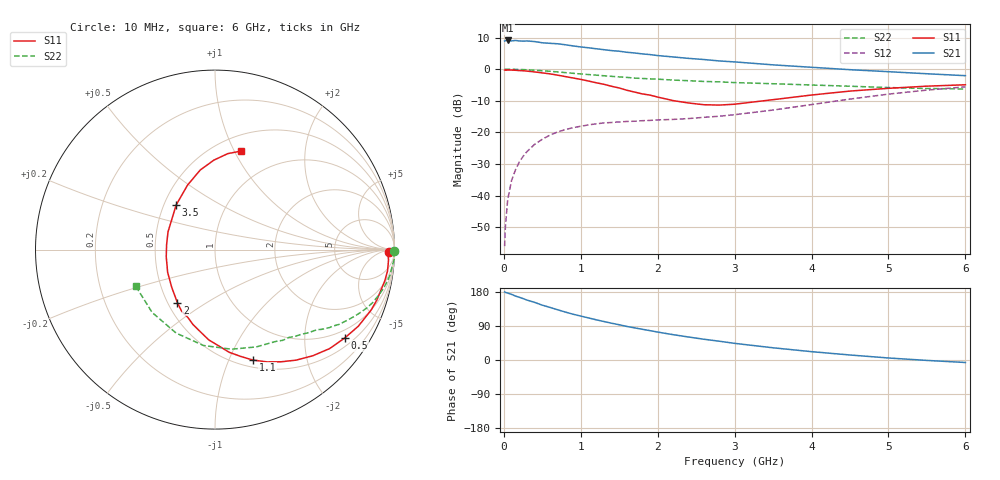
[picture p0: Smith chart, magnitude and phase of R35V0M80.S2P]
! SIEMENS Small Signal Semiconductors
! BFR181
! Si NPN RF Bipolar Junction Transistor in SOT23
! VCE = 5 V  IC = 0.8 mA
! Common Emitter S-Parameters:  May  1996
# GHz  S  MA  R  50
!  f  S11  S21  S12  S22
! GHz  MAG  ANG  MAG  ANG  MAG  ANG  MAG  ANG
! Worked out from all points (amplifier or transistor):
!   36 points, 10 MHz to 6 GHz, reference 50 ohm
!   highest |S21| = 9.1 dB at 50 MHz (marker M1)
!   |S21| within 3 dB of that: start of sweep to 1.329 GHz
!   unconditionally stable (mu >= 1): 2.149 GHz to 3.752 GHz
!   at 250 MHz: K = 0.15, MSG = 18.2 dB, |S12| = -27.6 dB
!   at 1.4 GHz: K = 0.70, MSG = 11.4 dB, |S12| = -16.8 dB
!   at 6 GHz: K = 0.89, MSG = 1.8 dB, |S12| = -5.6 dB
!   S11 on the Smith chart (normalised r, x): 10 MHz: 54, -24; 500 MHz: 0.74, -3.08; 1.1 GHz: 0.58, -1.23; 2 GHz: 0.56, -0.38; 3.5 GHz: 0.58, +0.32; 6 GHz: 0.66, +1.06
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0.01  0.9694 -0.8  2.783 179.6  0.0016 91.0  0.9982 -0.4
0.02  0.9635 -1.3  2.812 178.4  0.0032 85.2  0.9996 -0.8
0.05  0.9686 -3.4  2.844 176.6  0.0087 89.2  0.9981 -1.7
0.1  0.9685 -7.1  2.799 173.3  0.0174 85.6  0.999 -3.3
0.15  0.9619 -10.5  2.844 168.8  0.0255 82.4  0.9924 -5.1
0.2  0.9515 -13.8  2.795 165.6  0.034 80.7  0.9886 -6.7
0.3  0.9327 -21.2  2.793 158.2  0.0498 76.0  0.9782 -9.9
0.4  0.9056 -28.1  2.733 152.1  0.0649 71.7  0.9633 -13.0
0.5  0.8745 -34.3  2.613 144.7  0.0782 67.6  0.9445 -15.9
0.7  0.8045 -47.3  2.521 132.5  0.102 60.0  0.9054 -21.1
0.8  0.7641 -53.7  2.431 126.5  0.1111 56.5  0.8828 -23.4
1.1  0.6504 -71.1  2.179 111.1  0.1317 49.0  0.8226 -29.4
1.3  0.5776 -82.1  2.034 101.6  0.1415 45.4  0.7877 -32.6
1.6  0.4645 -100.2  1.849 88.5  0.1495 42.0  0.7418 -36.8
2  0.3625 -125.3  1.641 73.7  0.158 41.1  0.6954 -41.8
2.2  0.3192 -139.2  1.561 66.9  0.1609 42.0  0.6731 -44.6
2.6  0.2745 -171.7  1.422 54.8  0.1736 44.8  0.6398 -49.9
3  0.2798 159.4  1.303 43.9  0.191 48.1  0.6139 -56.4
3.5  0.33 130.9  1.17 32.2  0.2262 50.8  0.5891 -67.0
4.5  0.4511 100.5  0.982 13.2  0.3371 48.4  0.5381 -96.9
5.5  0.5395 82.4  0.847 -1.1  0.4676 36.1  0.4954 -135.0
6  0.5674 75.3  0.79 -6.6  0.5256 28.0  0.4866 -155.3
